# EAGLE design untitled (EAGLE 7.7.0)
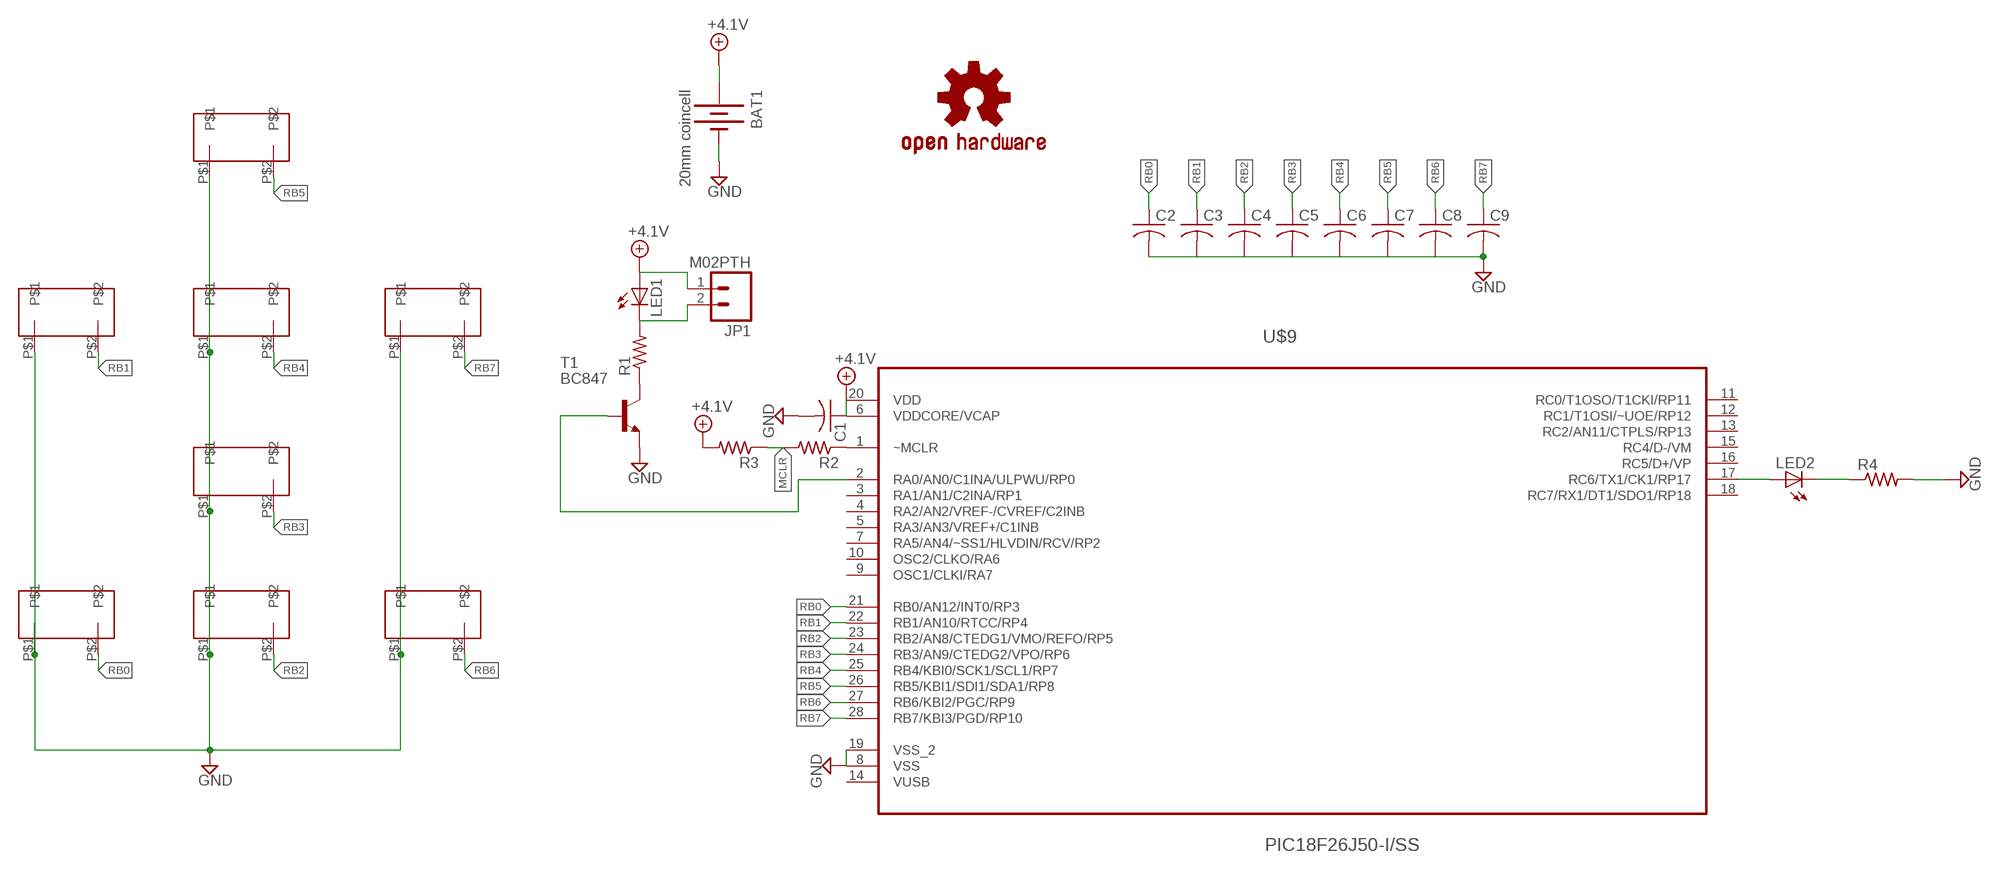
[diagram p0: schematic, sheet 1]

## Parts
BAT1  20mm coincell  BATTERY20MM_4LEGS  [BATTCON_20MM_4LEGS]
C1  C-USC1206  [C1206]
C2  C-USC1206  [C1206]
C3  C-USC1206  [C1206]
C4  C-USC1206  [C1206]
C5  C-USC1206  [C1206]
C6  C-USC1206  [C1206]
C7  C-USC1206  [C1206]
C8  C-USC1206  [C1206]
C9  C-USC1206  [C1206]
JP1  M02PTH  [1X02]
LED1  LED5MM  [LED5MM]
LED2  LEDCHIPLED_1206  [CHIPLED_1206]
LOGO1  OSHW-LOGOM  [OSHW-LOGO-M]
R1  R-US_R0603  [R0603]
R2  R-US_R0603  [R0603]
R3  R-US_R0603  [R0603]
R4  R-US_R0603  [R0603]
T1  BC847  [SOT23]
U$1  CONDUCTIVE_PAD  [CONDUCTIVE_PAD]
U$2  CONDUCTIVE_PAD  [CONDUCTIVE_PAD]
U$3  CONDUCTIVE_PAD  [CONDUCTIVE_PAD]
U$4  CONDUCTIVE_PAD  [CONDUCTIVE_PAD]
U$5  CONDUCTIVE_PAD  [CONDUCTIVE_PAD]
U$6  CONDUCTIVE_PAD  [CONDUCTIVE_PAD]
U$7  CONDUCTIVE_PAD  [CONDUCTIVE_PAD]
U$9  PIC18F26J50-I/SS  [SOP65P780X200-28N]
U$10  CONDUCTIVE_PAD  [CONDUCTIVE_PAD]

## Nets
+4.1V: BAT1.1(+) BAT1.3(+) BAT1.P$1(+) BAT1.P$2(+) C1.1 JP1.1 LED1.A R3.2 U$9.6(VDDCORE/VCAP) U$9.20(VDD)
GND: BAT1.2(-) C1.2 C2.2 C3.2 C4.2 C5.2 C6.2 C7.2 C8.2 C9.2 R4.2 T1.2(E) U$1.P$1 U$2.P$1 U$3.P$1 U$4.P$1 U$5.P$1 U$6.P$1 U$7.P$1 U$9.8(VSS) U$9.19(VSS_2) U$10.P$1
MCLR: R2.2 R3.1
N$1: JP1.2 LED1.K(C) R1.2
N$2: R1.1 T1.3(C)
N$3: T1.1(B) U$9.2(RA0/AN0/C1INA/ULPWU/RP0)
N$5: R2.1 U$9.1(~MCLR)
N$6: LED2.A U$9.17(RC6/TX1/CK1/RP17)
N$9: LED2.C R4.1
RB0: C2.1 U$5.P$2 U$9.21(RB0/AN12/INT0/RP3)
RB1: C3.1 U$3.P$2 U$9.22(RB1/AN10/RTCC/RP4)
RB2: C4.1 U$6.P$2 U$9.23(RB2/AN8/CTEDG1/VMO/REFO/RP5)
RB3: C5.1 U$4.P$2 U$9.24(RB3/AN9/CTEDG2/VPO/RP6)
RB4: C6.1 U$1.P$2 U$9.25(RB4/KBI0/SCK1/SCL1/RP7)
RB5: C7.1 U$9.26(RB5/KBI1/SDI1/SDA1/RP8) U$10.P$2
RB6: C8.1 U$7.P$2 U$9.27(RB6/KBI2/PGC/RP9)
RB7: C9.1 U$2.P$2 U$9.28(RB7/KBI3/PGD/RP10)
Unconnected: U$9.3(RA1/AN1/C2INA/RP1) U$9.4(RA2/AN2/VREF-/CVREF/C2INB) U$9.5(RA3/AN3/VREF+/C1INB) U$9.7(RA5/AN4/~SS1/HLVDIN/RCV/RP2) U$9.9(OSC1/CLKI/RA7) U$9.10(OSC2/CLKO/RA6) U$9.11(RC0/T1OSO/T1CKI/RP11) U$9.12(RC1/T1OSI/~UOE/RP12) U$9.13(RC2/AN11/CTPLS/RP13) U$9.15(RC4/D-/VM) U$9.16(RC5/D+/VP) U$9.18(RC7/RX1/DT1/SDO1/RP18)

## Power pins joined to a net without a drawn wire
VUSB: U$9.14(VUSB)

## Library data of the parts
BAT1 = SparkFun-Electromechanical:BATTERY: Battery Holders; PROD_ID: BATT-10373
C1-C9 = rcl:C-US: CAPACITOR, American symbol
JP1 = SparkFun-Connectors:M02: Standard 2-pin 0.1" header. Use with
LED1 LED2 = led:LED: LED
LOGO1 = SparkFun-Aesthetics:OSHW-LOGO: Open Source Hardware Logo This logo indicates the piece of hardware it is found on incorporates a OSHW license and/or adheres to the definition of open source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
R1-R4 = rcl:R-US_: RESISTOR, American symbol
T1 = transistor-neu-to92:BC847: NPN TRANSISTOR
U$1-U$7 U$10 = CONDUCTIVE_PAD:CONDUCTIVE_PAD
U$9 = Microchip_By_element14_Batch_1:PIC18F26J50-I/SS: Low-Power High-Performance Microcontrollers; MPN: PIC18F26J50-I/SS; OC_FARNELL: 1706310; OC_NEWARK: 98M1806; PACKAGE: SSOP-28; SUPPLIER: Microchip

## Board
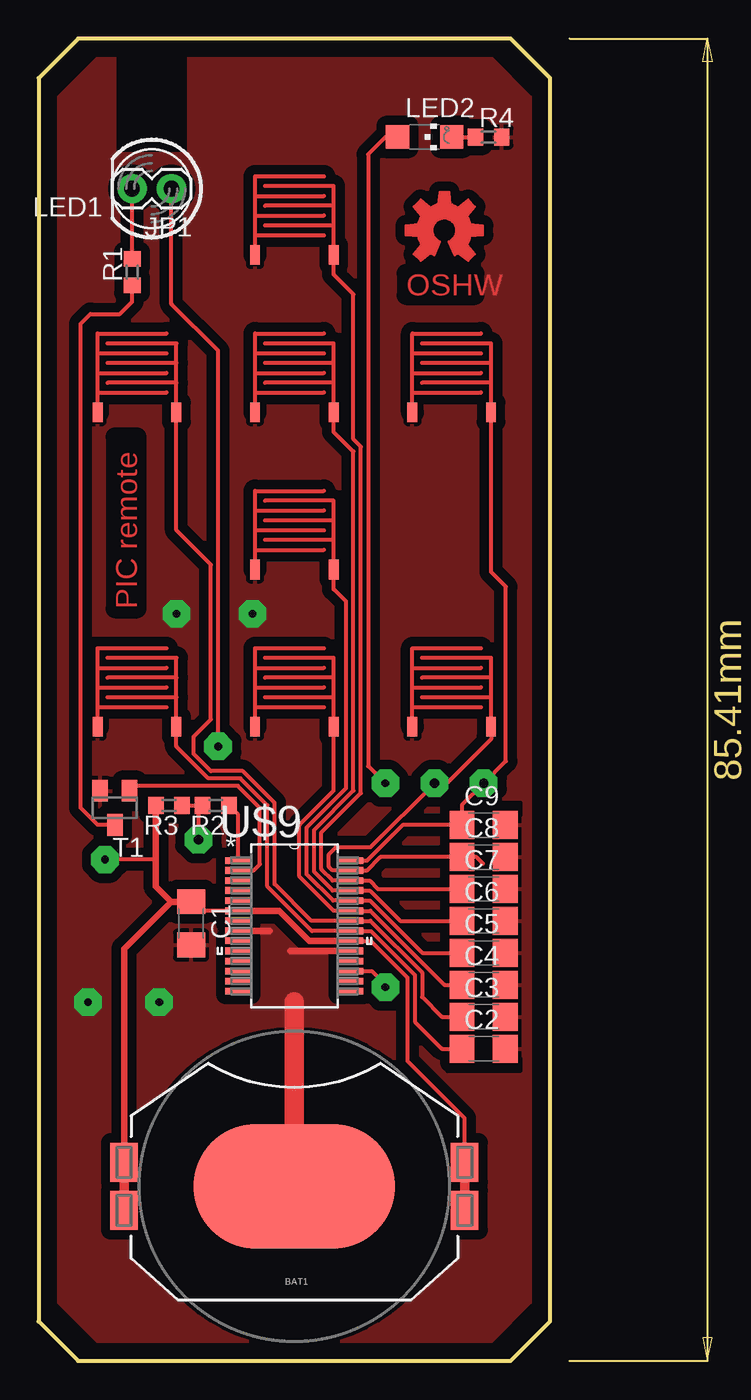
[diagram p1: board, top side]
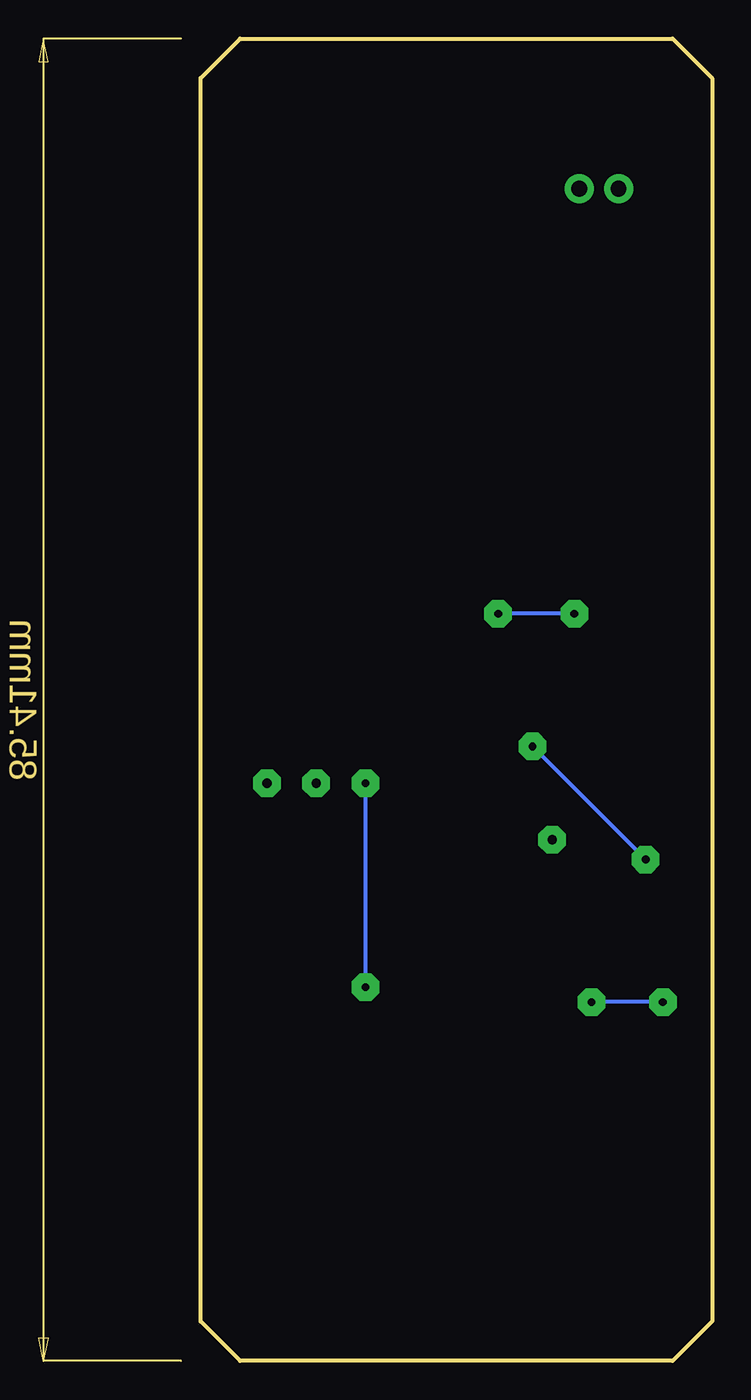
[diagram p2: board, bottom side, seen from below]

Size 43.48 x 85.41 mm. Coordinates in mm from the lower left corner, seen from the top.
Outline: 30.48,85.41 2.54,85.41 0,82.87 0,2.54 2.54,0 30.48,0 33.02,2.54 33.02,82.87 30.48,85.41
Copper layers (1*16): Top 0.035mm / dielectric 1.5mm / Bottom 0.035mm
Design rules "default *": minimum track width 10mil, minimum drill 24mil, track to track 8mil, track to pad 8mil, pad to pad 8mil, via to via 8mil, smd to smd 8mil, copper to edge 40mil, drill to drill 8mil, minimum pad ring 10mil, minimum via ring 8mil, stop-mask expansion 4mil, vias tented up to drill 0mil, thermal gap 10mil

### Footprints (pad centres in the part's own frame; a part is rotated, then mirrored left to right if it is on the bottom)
BATTCON_20MM_4LEGS = smd 1.778 x 2.54: 1 -11,1.55; 3 11,1.55; P$1 -11,-1.55; P$2 11,-1.55 | smd 13 x 8: 2 0,0
C1206 = smd 1.6 x 1.8: 1 -1.4,0; 2 1.4,0
1X02 = drill 1.016 pad 1.88: 1 0,0; 2 2.54,0
LED5MM = drill 0.813 octagon: A -1.27,0; K 1.27,0
CHIPLED_1206 = smd 1.5 x 1.5: A 0,-1.75; C 0,1.75
R0603 = smd 1 x 1.1: 1 -0.85,0; 2 0.85,0
SOT23 = smd 1 x 1.4: 1 -0.95,-1.1; 2 0.95,-1.1; 3 0,1.1
CONDUCTIVE_PAD = smd 0.635 x 1.27: P$1 -2.54,-2.54; P$2 2.54,-2.54
SOP65P780X200-28N = smd 1.651 x 0.432: 1 -3.632,4.216; 2 -3.632,3.581; 3 -3.632,2.921; 4 -3.632,2.286; 5 -3.632,1.626; 6 -3.632,0.965; 7 -3.632,0.33; 8 -3.632,-0.33; 9 -3.632,-0.965; 10 -3.632,-1.626; 11 -3.632,-2.286; 12 -3.632,-2.921; 13 -3.632,-3.581; 14 -3.632,-4.216; 15 3.632,-4.216; 16 3.632,-3.581; 17 3.632,-2.921; 18 3.632,-2.286; 19 3.632,-1.626; 20 3.632,-0.965; 21 3.632,-0.33; 22 3.632,0.33; 23 3.632,0.965; 24 3.632,1.626; 25 3.632,2.286; 26 3.632,2.921; 27 3.632,3.581; 28 3.632,4.216

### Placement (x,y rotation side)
BAT1  16.51,11.27 180 top
C1  9.84,28.26 270 top
C2  28.73,20.16 0 top
C3  28.73,22.23 0 top
C4  28.73,24.29 0 top
C5  28.73,26.35 0 top
C6  28.73,28.42 0 top
C7  28.73,30.48 0 top
C8  28.73,32.54 0 top
C9  28.73,34.61 0 top
JP1  8.57,75.72 180 top
LED1  7.3,75.72 180 top
LED2  24.92,79.06 270 top
LOGO1  26.19,73.03 0 top
R1  6.03,70.33 90 top
R2  11.43,35.88 180 top
R3  8.41,35.88 180 top
R4  29.05,79.06 0 top
T1  4.92,35.72 180 top
U$1  16.51,63.82 0 top
U$2  26.67,63.82 0 top
U$3  6.35,63.82 0 top
U$4  16.51,53.66 0 top
U$5  6.35,43.5 0 top
U$6  16.51,43.5 0 top
U$7  26.67,43.5 0 top
U$9  16.51,28.1 0 top
U$10  16.51,73.98 0 top

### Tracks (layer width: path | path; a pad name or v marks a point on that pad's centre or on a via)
+4.1V  (via drill 0.5 pad 1.78)
  Top 0.254: U$9.6 10.44,29.06 C1.1 | U$9.20 21.44,27.13 23.81,24.77 23.81,19.37 27.51,15.67 BAT1.P$1 | 7.56,32.38 v4.29,32.38 | v11.59,39.69 11.59,65.25 8.57,68.26 JP1.1
  Top 0.406: BAT1.P$2 5.51,26.62 8.54,29.66 | R3.2 7.56,32.38 7.56,30.64 8.54,29.66 | U$9.20 17.48,27.13 15.54,29.06 U$9.6 | 8.54,29.66 C1.1
  Top 0.61: BAT1.1 BAT1.P$1 | BAT1.3 BAT1.P$2
  Bottom 0.254: v11.59,39.69 v4.29,32.38
GND  (via drill 0.5 pad 1.78)
  Top 0.406: U$9.8 14.94,27.77 | 16.23,26.47 U$9.19
  Top 1.27: BAT1.2 16.51,23.18
  Bottom 0.254: v3.17,23.18 v7.78,23.18 | v8.89,48.26 v13.81,48.26
  pour Top (isolate 0.61): 3.81,1.27 29.21,1.27 31.75,3.81 31.75,81.6 29.21,84.14 9.68,84.14 9.68,77.95 4.92,77.95 4.92,84.14 3.81,84.14 1.27,81.6 1.27,3.81
MCLR  (via drill 0.6 pad 1.78)
  Top 0.254: R3.1 R2.2 10.32,35.77 v10.32,33.66
N$1
  Top 0.254: R1.2 JP1.2
N$2
  Top 0.254: T1.3 3.8,34.62 2.7,35.72 2.7,66.99 3.33,67.63 5.24,67.63 6.03,68.42 R1.1
N$3
  Top 0.254: U$9.2 13.9,31.68 14.29,32.07 14.29,35.72 12.86,37.15 5.72,37.15 T1.1
N$5
  Top 0.254: U$9.1 12.88,35.28 R2.1
N$6  (via drill 0.5 pad 1.78)
  Top 0.254: v22.38,37.31 21.27,38.42 21.27,77.95 22.38,79.06 LED2.A | U$9.17 21.5,25.18 22.38,24.29 v22.38,24.13
  Bottom 0.254: v22.38,37.31 v22.38,24.13
N$7
  cutout Top: 6.35,11.43 6.35,11.11 arc90 16.35,1.11 16.67,1.11 arc90 26.67,11.11 26.67,11.43 arc90 16.67,21.43 16.35,21.43 arc90
N$8
  cutout Top: 6.03,15.72 10.95,19.21 22.07,19.21 26.99,15.72 26.99,6.67 23.97,3.97 9.05,3.97 6.03,6.67
N$9
  Top 0.254: LED2.C R4.1
N$10
  cutout Top: 26.35,36.04 26.35,18.73 31.11,18.73 31.11,19.53 30.64,19.53 30.64,35.24 31.11,35.24 31.11,36.04
RB0
  Top 0.254: U$5.P$2 8.89,39.69 10.95,37.62 13.02,37.62 14.76,35.88 14.76,30.64 17.63,27.77 U$9.21 21.44,27.77 24.29,24.92 24.29,21.91 26.04,20.16 C2.1
RB1
  Top 0.254: U$3.P$2 8.89,53.66 11.11,51.44 11.11,41.43 10,40.32 10,39.21 11.11,38.1 13.18,38.1 15.24,36.04 15.24,30.8 17.61,28.43 U$9.22 21.42,28.43 24.77,25.08 24.77,23.5 26.04,22.23 C3.1
RB2
  Top 0.254: U$6.P$2 19.05,36.83 16.83,34.61 16.83,31.27 19.04,29.06 U$9.23 21.42,29.06 26.19,24.29 C4.1
RB3
  Top 0.254: U$4.P$2 19.05,49.85 19.84,49.05 19.84,36.99 17.3,34.45 17.3,31.43 19.01,29.72 U$9.24 21.39,29.72 24.77,26.35 C5.1
RB4
  Top 0.254: U$1.P$2 19.05,60.01 20.32,58.74 20.32,36.83 17.78,34.29 17.78,31.59 18.99,30.39 U$9.25 21.37,30.39 23.34,28.42 C6.1
RB5
  Top 0.254: U$10.P$2 19.05,70.17 20.32,68.9 20.32,59.53 20.8,59.05 20.8,36.67 18.26,34.13 18.26,31.75 18.99,31.02 U$9.26 21.37,31.02 21.91,30.48 C7.1
RB6  (via drill 0.6 pad 1.78)
  Top 0.254: U$7.P$2 29.21,40.16 26.35,37.31 v25.56,37.31 21.43,33.18 19.21,33.18 18.73,32.7 18.73,31.91 18.96,31.68 U$9.27 21.2,31.68 22.07,32.54 C8.1 28.26,32.54 28.68,32.12
RB7  (via drill 0.6 pad 1.78)
  Top 0.254: U$2.P$2 29.21,50.96 30.16,50.01 30.16,38.73 v28.73,37.31 27.33,35.91 C9.1 23.5,34.61 21.2,32.31 U$9.28

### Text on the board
Top: OSHW | PIC remote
